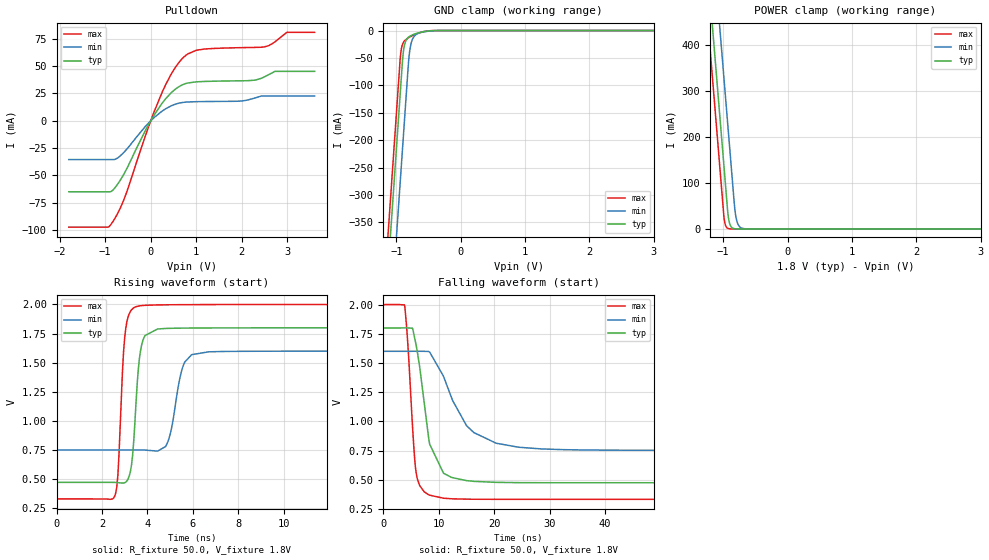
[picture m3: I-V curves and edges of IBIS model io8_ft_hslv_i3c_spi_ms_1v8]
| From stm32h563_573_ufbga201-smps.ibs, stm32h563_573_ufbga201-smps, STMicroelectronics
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[Model]   io8_ft_hslv_i3c_spi_ms_1v8
Model_type I/O_open_drain
Polarity   Non-Inverting
Enable   Active-Low
| CAP_THRESHOLD on pad IOFT is "UDTCAPC" :
| Rising=20.0% of vddiom   Falling=80.0% of vddiom
| C_comp min and max val. don't necessarily correlate with the min and max pvt
| but are the smallest and greatest pad capacitance found.
| var   typ   min   max
C_comp   3.75311pF  3.69067pF  3.87717pF
|C_comp_pulldown   3.75311pF  3.69067pF  3.87717pF
Vinl = 800.0mV
Vinh = 1.0V
Vmeas = 900.0mV   | Reference voltage for timing measurements
Cref  = 50.0pF   | Timing specification test load capacitance value
Rref  = 1.0MOhm   | Timing specification test load resistance value
Vref  = 990.0mV   | Timing specification test load voltage
[Model Spec]
| TIME_THRESHOLD on pin ZII2CV11 is "CMOS" :
| Rising=40.0% of vdd   Falling=60.0% of vdd
Vinl 703.80000mV 631.80000mV 784.80000mV
Vinh 1.06220V 937.20000mV 1.16620V
| variable   typ   min   max
[Temperature Range] 25.0 125.0 -40.0
| variable   typ   min   max
[Voltage Range] 1.8V 1.6V 2.0V
| variable   typ   min   max
[POWER Clamp Reference] 1.8V 1.6V 2.0V
| variable   typ   min   max
[GND Clamp Reference] 0V 0V 0V
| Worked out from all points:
|   slope of the pulldown table from 0 to 0.27 V, typ, clamps not added: 15.8 ohm
|   GND clamp passes 1 mA (typ) near -0.52 V on its own axis
|   POWER clamp passes 1 mA (typ) near -0.84 V on its own axis
|   rising waveform, R_fixture 50.0, V_fixture 1.8V: 20-80 % time 286ps typ, 461ps min, 244ps max; typ from 0.474 V to 1.8 V
|   falling waveform, R_fixture 50.0, V_fixture 1.8V: 20-80 % time 2.68ns typ, 5.61ns min, 1.27ns max; typ from 1.8 V to 0.474 V
[POWER Clamp]
-1.8V     1.518A     1.709A     1.407A
-1.23V    548.8mA    740.2mA    437.5mA
-1.16V    429.8mA    621.2mA    318.5mA
-1.05V    242.8mA    434.2mA    131.5mA
-980mV    123.8mA    315.2mA    17.95mA
-930mV    38.81mA    230.2mA    1.49mA
-910mV    17.82mA    196.2mA    550.8uA
-890mV    8.18mA     162.2mA    203.5uA
-810mV    363.5uA    33.6mA     3.797uA
-770mV    76.62uA    10.47mA    518.8nA
-710mV    7.416uA    1.822mA    26.34nA
3.6V      0A         0A         0A
[GND Clamp]
-1.8V     -1.579A    -1.74A     -1.515A
-1.24V    -627.3mA   -788.3mA   -562.7mA
-1.05V    -304.3mA   -465.3mA   -239.7mA
-940mV    -117.3mA   -278.3mA   -52.69mA
-930mV    -100.3mA   -261.3mA   -40.52mA
-900mV    -50.11mA   -210.3mA   -24.23mA
-880mV    -30.95mA   -176.3mA   -20.02mA
-810mV    -12.18mA   -57.97mA   -13.23mA
-780mV    -9.807mA   -29.1mA    -11.19mA
-690mV    -5.41mA    -7.142mA   -6.184mA
-420mV    -170.4uA   -446.1uA   -81.94uA
3.6V      5.755nA    953.4nA    228.2pA
| variable   typ   min   max
[Pullup Reference] 1.8V 1.6V 2.0V
| variable   typ   min   max
[Pulldown Reference] 0V 0V 0V
[Pulldown]
-1.8V     -65.02mA   -35.56mA   -97.42mA
-940mV    -65.02mA   -35.56mA   -97.42mA
-850mV    -64.17mA   -35.56mA   -93.49mA
-570mV    -47.32mA   -28.01mA   -70.04mA
-120mV    -9.088mA   -5.279mA   -14.07mA
250mV     16.04mA    8.832mA    26.05mA
550mV     29.17mA    15.25mA    49.41mA
780mV     34.17mA    17.07mA    60.14mA
1.18V     35.97mA    17.56mA    65.65mA
2.49V     40mA       22.62mA    67.56mA
2.99V     45.21mA    22.62mA    80.94mA
3.6V      45.21mA    22.62mA    80.94mA
[Ramp]
dV/dt_r 795.76525mV/283.81834ps 508.94533mV/459.71097ps 1.00097V/239.63637ps
dV/dt_f 795.7872mV/2.30001ns 508.97859mV/5.41937ns 1.00099V/1.26668ns
R_load = 50.0
| Removed startup time: 0s 0s 0s  .
| Removed end time: 36.4ns.
[Rising Waveform]
R_fixture   = 50.0
V_fixture   = 1.8V
V_fixture_min = 1.6V
V_fixture_max = 2.0V
0s        473.7mV    751.7mV    331.7mV
2.55ns    473.1mV    751.8mV    350.6mV
2.7ns     471.3mV    751.8mV    532.2mV
3.05ns    475.9mV    751.8mV    1.799V
3.35ns    708.2mV    751.9mV    1.964V
3.6ns     1.444V     751.8mV    1.986V
4.8ns     1.794V     781.3mV    1.997V
5.6ns     1.797V     1.486V     1.998V
6.7ns     1.799V     1.594V     1.999V
36.4ns    1.8V       1.6V       2V
| Removed startup time: 0s 0s 0s  .
| Removed end time: 199.4ns.
[Falling Waveform]
R_fixture   = 50.0
V_fixture   = 1.8V
V_fixture_min = 1.6V
V_fixture_max = 2.0V
0s        1.8V       1.6V       2V
3.8ns     1.801V     1.6V       1.998V
5.25ns    1.796V     1.6V       961.8mV
5.85ns    1.666V     1.6V       581mV
6.55ns    1.466V     1.6V       449.3mV
8.35ns    804.5mV    1.593V     367.1mV
10.85ns   555.4mV    1.386V     341.3mV
16.3ns    485.8mV    904.2mV    332.5mV
28.5ns    474mV      763.5mV    331.7mV
199.4ns   473.7mV    751.7mV    331.7mV
